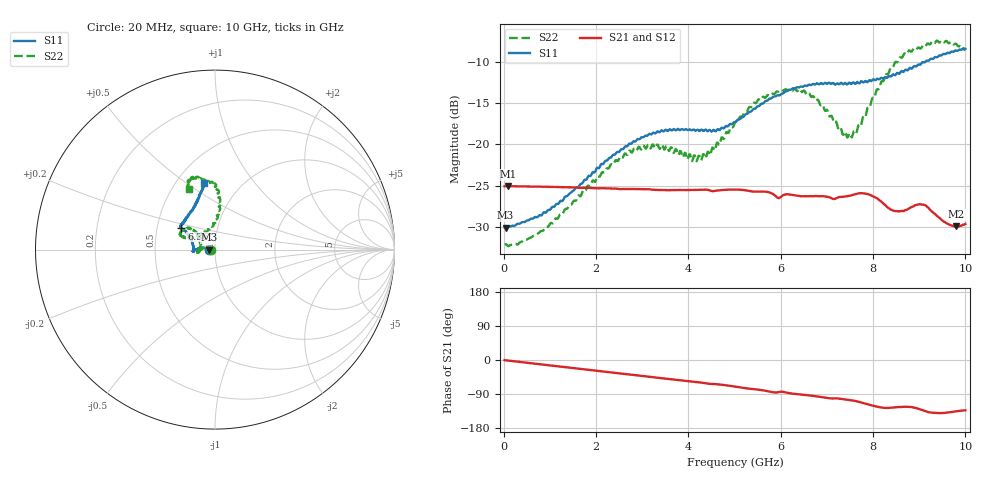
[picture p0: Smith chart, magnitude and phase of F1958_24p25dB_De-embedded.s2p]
! Integrated Device Technology
! Corporate Headquarters
! 6024 Silver Creek Valley Road
! San Jose, CA 95138  USA
! Phone:  1-408-284-8200
! Toll Free:  1-800-223-1366
! Webpage:  http://www.idt.com/
! Timing and RF Division
! 515 Groton Road, Suite 102
! Westford, MA 01886-6024
! Device:  F1958
! Description: 7-bit 0.25 dB Digital Step Attenuator
! Frequency:  0.001 -  6.000 GHz
! Package:  4x4 mm Thin QFN Plastic Package: 24 pin
! Ports:  2 RF, 12 DC
!  Pin  1  = D0
!  Pin  2  = VDD
!  Pin  3  = VMODE
!  Pin  4  = GND
!  Pin  5  = RF1  =  Port 1
!  Pin  6  = GND
!  Pin  7  = GND
!  Pin  8  = GND
!  Pin  9  = GND
!  Pin 10  = GND
!  Pin 11  = GND
!  Pin 12  = GND
!  Pin 13  = GND
!  Pin 14  = RF2  =  Port 2
!  Pin 15  = GND
!  Pin 16  = LE
!  Pin 17  = CLK
!  Pin 18  = DATA
!  Pin 19  = D6
!  Pin 20  = D5
!  Pin 21  = D4
!  Pin 22  = D3
!  Pin 23  = D2
!  Pin 24  = D1
! State:  97
! Atten State:  24.25 dB
! Voltage:  +3.30 Volts
! Current:  0.258 mA
! Data:  The device was measured on a F1958 evaluation board which has
!  individual transmission lines to the RF pins.  Data was collected
!  using a calibrated network analyzer.  The evaluation board was
!  de-embedded using Automatic Fixture Removal (AFR).
!  The reference plane is the edge of the package pin.
! Misc:
!  Action Tracker AT0419
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# GHz S dB R 50
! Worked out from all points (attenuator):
!   500 points, 20 MHz to 10 GHz, reference 50 ohm
!   highest |S21| = -25.05 dB at 100 MHz (marker M1); lowest = -29.9 dB at 9.8 GHz (marker M2)
!   lowest |S11| = -30.1 dB at 40 MHz (marker M3), VSWR 1.06, Z = 47 - j0.0443 ohm
!   |S11| at or under -10 dB: start of sweep to 9.137 GHz
!   |S22| runs from -32.3 to -7.5 dB; largest |S21 - S12| = 0.00032
!   S11 on the Smith chart (normalised r, x): 20 MHz: 0.94, -0.00; 6.36 GHz: 0.67, +0.17; 10 GHz: 0.68, +0.59
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0.02  -30.03 -178.9  -25.05 -0.4  -25.04 -0.3  -32.07 -178.9
0.04  -30.05 -179.1  -25.05 -0.6  -25.05 -0.6  -32.05 -178.4
0.1  -29.93 179.3  -25.05 -1.5  -25.05 -1.5  -32.30 -180.0
0.84  -28.43 171.3  -25.12 -12.1  -25.11 -12.1  -30.45 172.8
1.7  -24.75 171.3  -25.26 -24.1  -25.25 -24.1  -25.82 171.9
2.62  -20.31 177.2  -25.39 -36.8  -25.36 -36.8  -21.12 -179.1
3.36  -18.52 -175.6  -25.51 -47.2  -25.51 -47.4  -20.36 -169.3
4.24  -18.40 -179.1  -25.49 -59.1  -25.50 -59.1  -21.41 169.0
4.5  -18.46 175.0  -25.63 -63.2  -25.65 -63.3  -20.78 151.8
5.02  -17.32 160.7  -25.45 -70.4  -25.46 -70.4  -17.26 138.5
5.58  -15.09 150.4  -25.71 -79.4  -25.72 -79.4  -14.55 140.0
6.36  -13.10 147.8  -26.21 -90.3  -26.23 -90.3  -13.59 155.3
6.68  -12.77 146.3  -26.25 -94.3  -26.27 -94.3  -14.24 157.3
7.32  -12.59 141.0  -26.34 -103.0  -26.34 -102.9  -18.34 138.8
7.5  -12.60 137.9  -26.21 -105.6  -26.21 -105.6  -18.67 119.4
7.68  -12.56 135.0  -25.93 -109.9  -25.92 -109.9  -17.74 99.8
7.9  -12.36 128.5  -26.03 -117.3  -26.03 -117.4  -15.50 89.5
8.34  -11.76 118.6  -27.70 -126.4  -27.71 -126.6  -11.37 83.9
8.66  -11.26 112.9  -28.07 -123.7  -28.02 -123.7  -9.20 87.5
9.1  -10.11 106.8  -27.31 -133.2  -27.28 -133.4  -8.09 100.0
9.8  -8.67 100.3  -29.92 -135.6  -29.89 -135.5  -7.87 112.3
10  -8.46 99.5  -29.62 -132.9  -29.63 -132.7  -8.63 113.3
